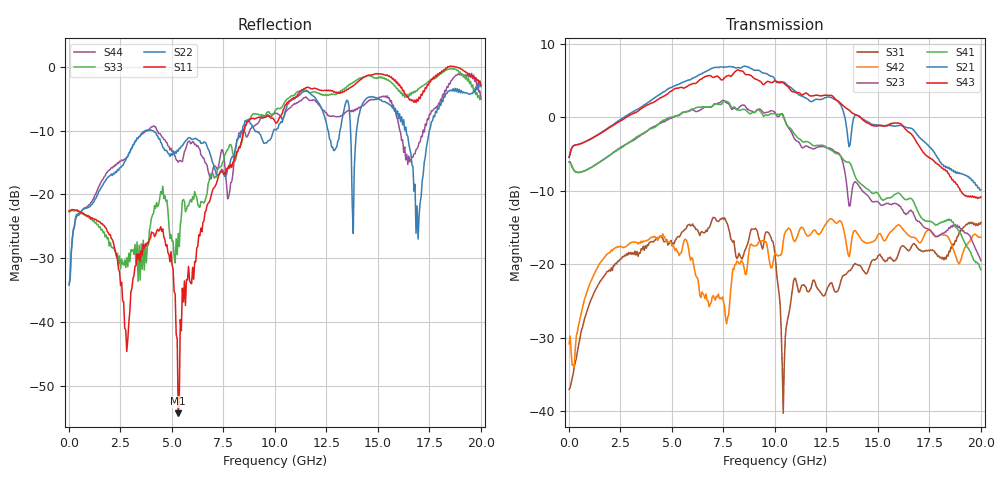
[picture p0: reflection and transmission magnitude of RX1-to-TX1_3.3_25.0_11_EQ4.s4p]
!Agilent Technologies,N5225A,MY51451112,A.09.50.13
!Agilent N5225A: A.09.50.13
!Date: Wednesday, January 31, 2018 11:03:29
!Correction: S11(Full 4 Port(1,2,3,4))
!S12(Full 4 Port(1,2,3,4))
!S13(Full 4 Port(1,2,3,4))
!S14(Full 4 Port(1,2,3,4))
!S21(Full 4 Port(1,2,3,4))
!S22(Full 4 Port(1,2,3,4))
!S23(Full 4 Port(1,2,3,4))
!S24(Full 4 Port(1,2,3,4))
!S31(Full 4 Port(1,2,3,4))
!S32(Full 4 Port(1,2,3,4))
!S33(Full 4 Port(1,2,3,4))
!S34(Full 4 Port(1,2,3,4))
!S41(Full 4 Port(1,2,3,4))
!S42(Full 4 Port(1,2,3,4))
!S43(Full 4 Port(1,2,3,4))
!S44(Full 4 Port(1,2,3,4))
!S4P File: Measurements: <S11,S12,S13,S14>,
!<S21,S22,S23,S24>,
!<S31,S32,S33,S34>,
!<S41,S42,S43,S44>:
# Hz S  RI  R 50
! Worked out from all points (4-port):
!   401 points, 10 MHz to 20 GHz, reference 50 ohm
!   strongest paths, dB at 10 MHz, 5.008 GHz, 10.01 GHz, 15 GHz, 20 GHz:
!     S43: -5.5, 3.7, 5.0, -1.1, -10.8
!     S21: -5.4, 4.1, 5.1, -1.1, -9.8
!     S41: -6.1, 0.0, 0.5, -10.3, -20.7
!     S23: -6.1, -0.1, 0.7, -11.5, -19.5
!     S42: -30.8, -17.3, -18.5, -16.0, -16.3
!     S31: -37.0, -17.5, -18.6, -18.8, -14.3
!   lowest |S11| = -54.2 dB at 5.307 GHz (marker M1), VSWR 1.00, Z = 50.1 + j0.142 ohm
!   |S11| at or under -10 dB: start of sweep to 8.504 GHz
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1e7  -0.0746 -0.00301  -0.000561 8.01e-05  0.0139 0.000825  0.000176 0.000336
     0.5361 0.00861  -0.0136 0.014  -0.4975 0.00304  0.0264 0.012
     0.014 0.000812  5.32e-05 0.000547  -0.073 -0.00385  -0.000297 0.000615
     -0.4979 0.00341  0.0259 0.0123  0.5337 0.00759  -0.0132 0.015
5.30735e9  0.00133 0.00141  0.0286 -0.00416  0.0906 0.1368  0.0296 -0.0138
           -0.7068 -1.52  0.1247 -0.1784  0.6369 0.8052  0.1217 0.0101
           0.0862 0.1283  0.0329 -0.000839  0.0419 0.0264  0.0406 -0.0101
           0.8479 0.5961  0.119 0.0146  -1.178 -1.053  0.0637 -0.1669
7.156425e9  -0.0161 0.12  0.0159 -0.0198  0.1307 0.0868  0.00163 -0.0335
            -2.192 0.1117  0.1245 -0.0698  1.198 -0.3207  0.0522 0.0241
            0.1654 0.111  0.0246 -0.0278  0.02 0.1347  0.00922 -0.0491
            0.9535 -0.7915  0.0602 -0.0064  -1.625 0.9845  0.11 -0.1201
8.8056e9  0.0126 0.3843  0.012 -0.0145  0.119 0.098  -0.0064 -0.0154
          -0.6675 2.056  -0.0925 0.347  0.1585 -1.099  0.0268 0.1297
          0.1289 0.1024  0.0014 -0.0235  0.0597 0.3884  -0.014 -0.0257
          -0.3313 -1.003  -0.000615 0.1361  0.4647 1.878  0.2577 0.1991
1.275362e10  0.2765 0.5822  -0.0385 -0.00669  0.0239 0.0634  -0.0319 0.00994
             1.196 -0.6541  0.1623 0.1695  -0.4753 0.3829  0.1899 0.1046
             0.0283 0.0694  -0.0307 -0.00843  0.4067 0.457  -0.0437 0.00153
             -0.1407 0.5792  0.1785 0.0967  0.3561 -1.366  0.2198 -0.343
1.665168e10  0.5223 0.1359  -0.0277 0.0163  -0.0577 0.1085  -0.00306 0.0372
             -0.7495 -0.3771  0.0085 0.1712  0.156 0.168  0.0928 0.1106
             -0.0621 0.1185  -0.0261 0.00428  0.6049 -0.1772  -0.0084 0.0369
             0.2724 -0.0536  0.1069 0.109  -0.5242 0.5519  -0.1116 -0.1609
2e10  0.7125 0.0618  0.0231 0.035  -0.0792 0.1677  0.0345 0.0207
      -0.0541 0.3175  0.6936 0.0763  0.0838 -0.0648  0.1522 0.0429
      -0.0817 0.1738  0.0063 0.0478  0.5663 -0.0299  0.0477 0.0206
      -0.0335 -0.0856  0.146 0.0458  0.2449 0.1503  -0.1528 -0.5338
